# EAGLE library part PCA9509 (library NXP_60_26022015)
The PCA9509 is a level translating I2C-bus/SMBus repeater with two voltage supplies that enables processor low voltage 2-wire serial bus to interface with standard I2C-bus or SMBus I/O. AAL Eindhoven MK
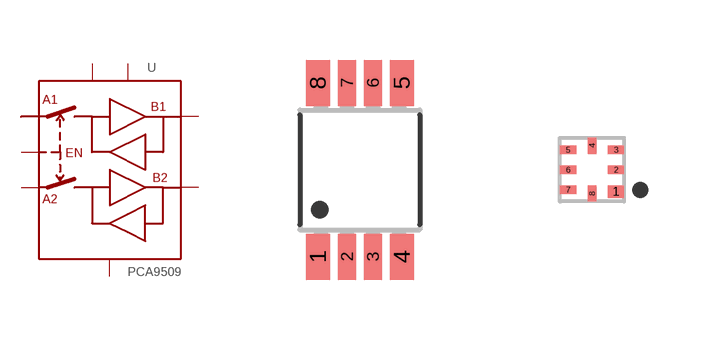
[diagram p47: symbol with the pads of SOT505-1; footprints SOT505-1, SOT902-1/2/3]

Designator prefix U

## PCA9509DP  [SOT505-1]
1  VCC(A)  pwr
2  A1
3  A2
4  GND  pwr
5  EN  in
6  B2
7  B1
8  VCC(B)  pwr

## PCA9509GM  [SOT902-1/2/3]
Pads as for SOT505-1

## PCA9509D  [SOT96-1]
Pads as for SOT505-1

## Footprint SOT505-1 (pad centres in mm)
SOT505-1 TSSOP8: plastic thin shrink small outline package; 8 leads; body width 3 mm JEDEC: -- IEC: --
smd 0.6 x 1.15: 1 -1.05,-2.175; 4 1.05,-2.175; 5 1.05,2.175; 8 -1.05,2.175
smd 0.45 x 1.15: 2 -0.325,-2.175; 3 0.325,-2.175; 6 0.325,2.175; 7 -0.325,2.175

## Footprint SOT902-1/2/3 (pad centres in mm)
SOT902-1/2/3 XQFN8U: plastic extremely thin quad flat package; no leads; 8 terminals; UTLP based; body 1.6 x 1.6 x 0.5 mm JEDEC: -- IEC: ---
smd 0.4 x 0.32: 1 0.6,-0.55
smd 0.4 x 0.22: 2 0.6,0; 3 0.6,0.5; 5 -0.6,0.5; 6 -0.6,0; 7 -0.6,-0.5
smd 0.22 x 0.4: 4 0,0.6; 8 0,-0.6

## Footprint SOT96-1 (pad centres in mm)
SOT96-1 SO8: plastic small outline package; 8 leads; body width 3.9 mm JEDEC: MS-012 IEC: 076E03
smd 0.6 x 1.3: 1 -1.905,-2.65; 2 -0.635,-2.65; 3 0.635,-2.65; 4 1.905,-2.65; 5 1.905,2.65; 6 0.635,2.65; 7 -0.635,2.65; 8 -1.905,2.65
